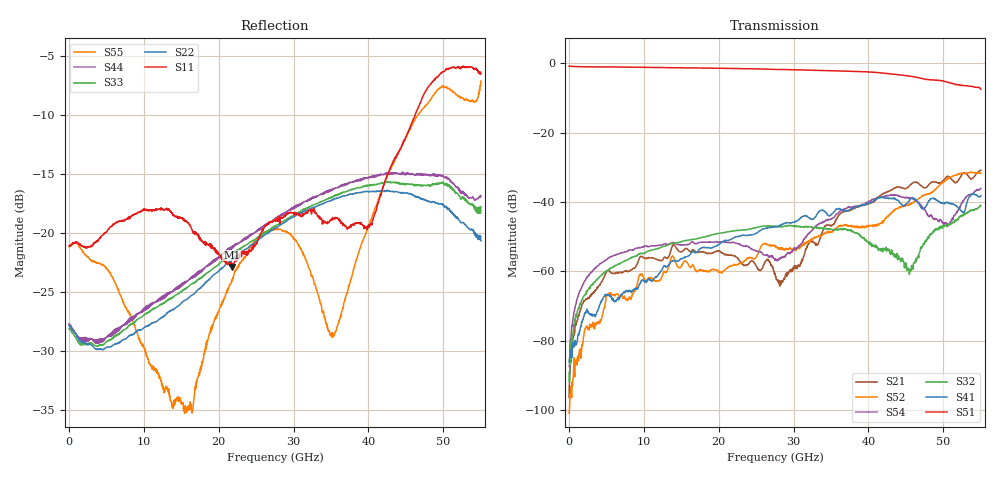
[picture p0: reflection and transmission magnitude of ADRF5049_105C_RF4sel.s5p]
! Device  : ADRF5049
! Description: Silicon SP4T Switch Non-Reflective
! Frequency:  9kHz -  45 GHz
! Ports:
!  RFC = Port 1
!  RF1 = Port 2
!  RF2 = Port 3
!	 RF3 = Port 4
!  RF4 = Port 5
! VSS  =  +3.30 Volts
! VDD  =  -3.30 Volts
! EN  =  0.00 Volts
! LS  =  0.00 Volts
! V1  =  3.30 Volts
! V2  =  3.30 Volts
! Data:  Data was collected using an calibrated 4 port network analyzer.
! Notes: Analog Devices supplies this data as a sample of measured data
!  for this product.  Your particular data for this product may vary.
!  Data was taken at 105 degrees C.
!  Analog Devices reserves the right to change this data at anytime.
# ghz S db R 50
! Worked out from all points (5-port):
!   1100 points, 50 MHz to 55 GHz, reference 50 ohm
!   strongest paths, dB at 50 MHz, 13.8 GHz, 27.55 GHz, 41.3 GHz, 55 GHz:
!     S51: -0.9, -1.3, -1.8, -2.7, -7.5
!     S41: -86.1, -57.1, -47.2, -38.9, -38.2
!     S32: -89.1, -52.0, -47.1, -54.0, -41.1
!     S54: -87.4, -51.8, -56.6, -38.7, -36.1
!     S52: -101.0, -55.7, -52.8, -46.4, -31.8
!     S21: -96.5, -52.8, -61.0, -38.7, -30.9
!   lowest |S11| = -22.9 dB at 21.75 GHz (marker M1), VSWR 1.15, Z = 54.9 + j5.72 ohm
!   |S11| at or under -10 dB: start of sweep to 46.22 GHz
